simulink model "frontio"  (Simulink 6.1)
settings: Solver=ode45  StartTime=0.0  StopTime=25.0  RelTol=1e-3
undefined symbols (not defined in the file or in its folder): Bit, frontio_netlist, Location, Lower, Width
libraries: xbsIndex_r3 x12, adlibrary2 x1

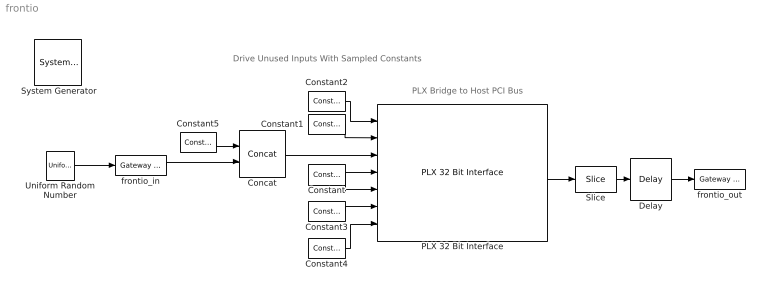
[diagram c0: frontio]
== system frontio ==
  note: Drive Unused Inputs With Sampled Constants
  note: PLX Bridge to Host PCI Bus
  " System Generator" : xbsIndex_r3/ System Generator  Tag=genX  xilinxfamily=Virtex2  part=xc2v4000  speed=-4  package=ff1152  synthesis_tool=XST  directory=./frontio_netlist  testbench=off  simulink_period=1  sysclk_period=10  incr_netlist=off  trim_vbits=Everywhere in SubSystem  dbl_ovrd=According to Block Masks  core_generation=According to Block Masks  run_coregen=off  deprecated_control=off  eval_field=0
  Concat : xbsIndex_r3/Concat  num_inputs=2  explicit_period=off  period=1  dbl_ovrd=off
  Constant : xbsIndex_r3/Constant  const=0  equ=P=C  arith_type=Boolean  n_bits=1  bin_pt=0  opselect=C  inp2=PCIN>>17  opr=+  inp1=P  carry=CIN  iostate=0  explicit_period=on  period=1  dbl_ovrd=off
  Constant1 : xbsIndex_r3/Constant  const=1  equ=P=C  arith_type=Boolean  n_bits=1  bin_pt=0  opselect=C  inp2=PCIN>>17  opr=+  inp1=P  carry=CIN  iostate=0  explicit_period=on  period=1  dbl_ovrd=off
  Constant2 : xbsIndex_r3/Constant  const=0  equ=P=C  arith_type=Unsigned  n_bits=32  bin_pt=0  opselect=C  inp2=PCIN>>17  opr=+  inp1=P  carry=CIN  iostate=0  explicit_period=on  period=1  dbl_ovrd=off
  Constant3 : xbsIndex_r3/Constant  const=0  equ=P=C  arith_type=Unsigned  n_bits=32  bin_pt=0  opselect=C  inp2=PCIN>>17  opr=+  inp1=P  carry=CIN  iostate=0  explicit_period=on  period=1  dbl_ovrd=off
  Constant4 : xbsIndex_r3/Constant  const=0  equ=P=C  arith_type=Unsigned  n_bits=34  bin_pt=0  opselect=C  inp2=PCIN>>17  opr=+  inp1=P  carry=CIN  iostate=0  explicit_period=on  period=1  dbl_ovrd=off
  Constant5 : xbsIndex_r3/Constant  const=0  equ=P=C  arith_type=Unsigned  n_bits=24  bin_pt=0  opselect=C  inp2=PCIN>>17  opr=+  inp1=P  carry=CIN  iostate=0  explicit_period=on  period=1  dbl_ovrd=off
  Delay : xbsIndex_r3/Delay  latency=1  reg_retiming=off  explicit_period=on  period=1  en=off  accept_only_valid=off  init_zero=on  dbl_ovrd=off  show_param=off
  PLX 32 Bit Interface : adlibrary2/ADM-XRC-II/PLX 32 Bit Interface  program='slave_write 0x40000 0xabcd1234;slave_read 0x40040'  clock_ratio=1.5
  Slice : xbsIndex_r3/Slice  mode=Lower Bit Location + Width  nbits=8  bit1=0  base1=MSB of Input  bit0=0  base0=LSB of Input  boolean_output=off  explicit_period=off  period=1  dbl_ovrd=off
  Uniform Random Number : UniformRandomNumber  SampleTime=0
  frontio_in : xbsIndex_r3/Gateway In  arith_type=Unsigned  n_bits=8  bin_pt=0  quantization=Truncate  overflow=Wrap  period=1  timing_constraint=None  locs_specified=on  LOCs={'B5','B4','C9','D9','B3','C2','E9','E8'}  needs_fixed_name=off  dbl_ovrd=off  show_param=off
  frontio_out : xbsIndex_r3/Gateway Out  output_type=Double  nbits=8  bin_pt=6  arith_type=Boolean  quantization=Truncate  overflow=Wrap  hdl_port=on  timing_constraint=None  locs_specified=on  LOCs={'B10','B9','C6','D6','D11','D10','J10','H11'}  needs_fixed_name=off  show_param=off
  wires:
  Constant/1 -> PLX 32 Bit Interface/4, PLX 32 Bit Interface/5
  Constant1/1 -> PLX 32 Bit Interface/2
  Constant2/1 -> PLX 32 Bit Interface/1
  Constant3/1 -> PLX 32 Bit Interface/6
  Constant4/1 -> PLX 32 Bit Interface/7
  PLX 32 Bit Interface/6 -> Slice/1
  Delay/1 -> frontio_out/1
  Slice/1 -> Delay/1
  frontio_in/1 -> Concat/2
  Concat/1 -> PLX 32 Bit Interface/3
  Constant5/1 -> Concat/1
  Uniform Random Number/1 -> frontio_in/1
